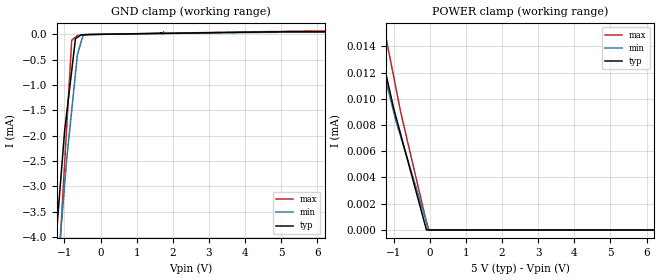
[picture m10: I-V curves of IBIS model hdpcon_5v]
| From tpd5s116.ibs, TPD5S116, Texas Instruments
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[Model]   hdpcon_5v
Model_type   Input
Vinl = .8
Vinh = 2
|   typ   min   max
|   (nom PVT)   (slow PVT)   (fast PVT)
C_comp   0.088p   0.0078p   0.872p
| Where nom  PVT is Nominal Process, 5V, 27C
|   Fast PVT is Strong Process,  5.5V, -40C
|   Slow PVT is Weak Process,   4.5V, 125C
[Voltage Range]   5   4.5   5.5
[Temperature Range]   27   125   -40
[Power Clamp Reference]   5   4.5   5.5
[GND Clamp Reference]   -0   -0   -0
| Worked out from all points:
|   GND clamp passes 1 mA (typ) near -0.85 V on its own axis
|   POWER clamp passes 1 mA (typ) near -5.00 V on its own axis
[GND Clamp]
|   Voltage   I(typ)   I(min)   I(max)
-5V       -143.7mA   -100.1mA   -185mA
-994.7mV  -1.911mA   -2.973mA   -2.554mA
-938.4mV  -1.568mA   -2.478mA   -1.853mA
-799.3mV  -721.6uA   -1.507mA   -118.3uA
-694.6mV  -85.04uA   -777.9uA   -55.02uA
-643.5mV  -61.21uA   -421.4uA   -24.07uA
-485.6mV  -8.399uA   -24.91uA   -10.34uA
-330.6mV  -5.889uA   -3.46uA    -3.887uA
1.743V    17.8uA     15.89uA    20.5uA
1.744V    17.81uA    15.9uA     48.61uA
1.744V    17.81uA    15.9uA     20.19uA
10V       51.2uA     41.49uA    66.03uA
[POWER Clamp]
|   Voltage   I(typ)   I(min)   I(max)
-5V       143.7mA    100.1mA    185mA
-994.7mV  9.244uA    8.979uA    11.66uA
-938.4mV  8.67uA     8.359uA    10.88uA
-799.3mV  7.249uA    7.092uA    8.936uA
-89.1mV   0A         622.6nA    585nA
-39.34mV  0A         169.5nA    0A
-20.73mV  0A         0A         0A
10V       0A         0A         0A
